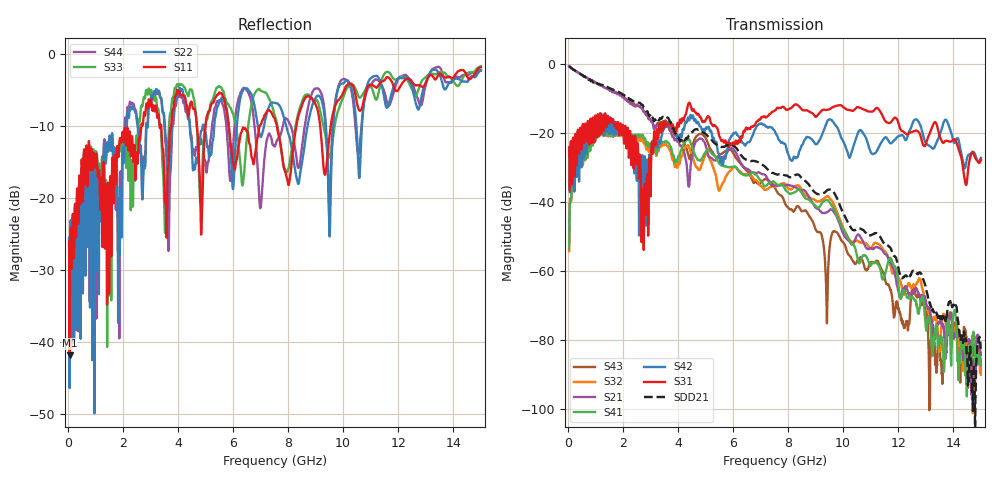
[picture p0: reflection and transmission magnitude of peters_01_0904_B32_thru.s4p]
# MHZ S RI R 50.00
! FREQ  S11  S12  S13  S14
!  S21  S22  S23  S24
!  S31  S32  S33  S34
!  S41  S42  S43  S44
!  REAL  IMAG  REAL  IMAG  REAL  IMAG  REAL  IMAG
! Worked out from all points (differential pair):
!   1496 points, 50 MHz to 15 GHz, reference 50 ohm
!   strongest paths, dB at 50 MHz, 3.79 GHz, 7.53 GHz, 11.27 GHz, 15 GHz:
!     S31: -24.3, -17.7, -13.5, -13.0, -27.9
!     S42: -24.4, -18.1, -19.8, -24.6, -27.3
!     S41: -53.5, -25.9, -34.6, -58.2, -85.7
!     S21: -0.7, -21.1, -35.3, -53.3, -83.9
!     S32: -54.3, -27.5, -35.6, -52.3, -90.1
!     S43: -0.7, -19.7, -36.1, -57.4, -87.9
!   taken as a pair (ports 1,3 in; 2,4 out), SDD21 dB: -0.7, -18.3, -32.0, -49.5, -82.3
!   lowest |S11| = -41.9 dB at 70 MHz (marker M1), VSWR 1.02, Z = 50.8 - j0.115 ohm
!   |S11| at or under -10 dB: start of sweep to 2.67 GHz; 5.847 GHz to 6.971 GHz (1.124 GHz wide, 17.5 % of centre); 7.589 GHz to 8.303 GHz (714.7 MHz wide, 8.99 % of centre)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
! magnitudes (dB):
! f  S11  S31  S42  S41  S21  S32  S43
! 50 MHz  -26.1  -24.3  -24.4  -53.5  -0.7  -54.3  -0.7
! 70 MHz  -41.9  -34.8  -35.1  -42.9  -0.9  -42.9  -0.9
! 1.59 GHz  -24.9  -17.0  -20.2  -19.8  -8.0  -19.9  -7.9
! 2.73 GHz  -9.8  -38.1  -29.0  -20.8  -13.4  -22.1  -13.5
! 4.37 GHz  -8.6  -11.9  -15.6  -21.8  -34.8  -23.6  -26.4
! 5.99 GHz  -15.0  -22.9  -20.6  -30.0  -24.6  -30.4  -25.7
! 15 GHz  -1.9  -27.9  -27.3  -85.7  -83.9  -90.1  -87.9
